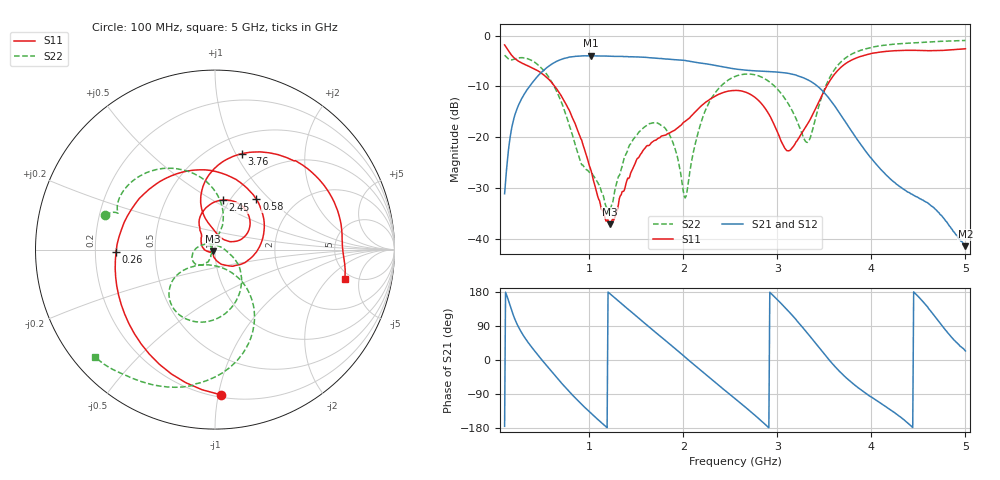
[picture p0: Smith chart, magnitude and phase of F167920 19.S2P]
!  2-Port S-parameters saved by WinCal
! VAR MeasName=S-Parameters (CALIBRATED_DATA) read from VNA (N5242A)
! VAR MeasDate=2016-11-22 9:56:07
! VAR NAME=F167920 19
! VAR FILENAME=F167920 19.S2P
! VAR DATE=2016-11-22 9:56:07
! VAR PHYS_PORTS=1,2
# Hz S DB R 50
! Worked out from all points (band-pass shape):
!   491 points, 100 MHz to 5 GHz, reference 50 ohm
!   highest |S21| = -3.96 dB at 1.02 GHz (marker M1); lowest = -41.5 dB at 5 GHz (marker M2)
!   |S21| within 3 dB of the highest: 507.7 MHz to 2.787 GHz (2.279 GHz wide, 138 % of centre)
!   lowest |S11| = -37.1 dB at 1.22 GHz (marker M3), VSWR 1.03, Z = 49 - j0.934 ohm
!   |S11| at or under -10 dB: 634.9 MHz to 3.523 GHz (2.888 GHz wide, 139 % of centre)
!   |S22| runs from -35.1 to -1.0 dB; largest |S21 - S12| = 0.0013
!   S11 on the Smith chart (normalised r, x): 100 MHz: 0.22, -1.01; 260 MHz: 0.29, -0.01; 580 MHz: 1.30, +0.84; 2.45 GHz: 0.93, +0.56; 3.76 GHz: 0.69, +1.06; 5 GHz: 4.36, -3.18
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1e8  -1.84 -87.8  -31.13 -175.0  -31.16 -175.0  -3.86 162.4
1.7e8  -3.75 -133.7  -18.74 134.4  -18.74 134.4  -4.78 159.4
2.6e8  -5.17 -178.6  -13.20 81.3  -13.19 81.3  -4.35 151.3
4.2e8  -6.59 113.0  -8.68 23.7  -8.68 23.7  -5.25 124.7
5.8e8  -8.81 50.5  -5.85 -24.8  -5.86 -24.8  -8.50 96.5
7.6e8  -13.74 -13.2  -4.36 -76.0  -4.36 -76.0  -15.96 73.8
9.2e8  -20.58 -63.5  -3.97 -117.1  -3.97 -117.1  -25.44 97.1
1.02e9  -26.60 -94.1  -3.96 -140.9  -3.97 -140.9  -26.98 122.0
1.22e9  -37.14 -136.7  -4.06 174.9  -4.06 174.9  -34.66 -163.8
1.44e9  -27.09 -166.7  -4.16 128.6  -4.16 128.6  -21.32 -123.3
1.74e9  -20.15 141.4  -4.49 65.8  -4.49 65.8  -17.35 -161.0
1.89e9  -18.79 130.9  -4.70 34.8  -4.71 34.8  -21.06 167.4
2.02e9  -16.88 125.8  -4.90 7.4  -4.90 7.4  -31.97 74.7
2.21e9  -13.55 111.7  -5.49 -32.1  -5.49 -32.1  -15.91 -34.2
2.45e9  -11.06 81.1  -6.25 -81.7  -6.26 -81.8  -9.13 -77.8
2.55e9  -10.77 67.1  -6.55 -101.9  -6.57 -101.9  -8.05 -92.8
2.95e9  -16.89 20.9  -7.10 171.5  -7.11 171.6  -9.61 -139.8
3.12e9  -22.68 58.1  -7.44 128.4  -7.45 128.5  -13.52 -146.7
3.37e9  -15.76 105.4  -9.18 55.6  -9.18 55.6  -18.89 -66.0
3.76e9  -5.11 74.4  -17.99 -52.9  -18.01 -52.9  -3.96 -79.2
4.19e9  -3.05 31.3  -28.01 -129.4  -28.03 -128.8  -1.78 -110.5
5e9  -2.59 -12.7  -41.46 23.9  -41.53 24.6  -0.95 -138.3
